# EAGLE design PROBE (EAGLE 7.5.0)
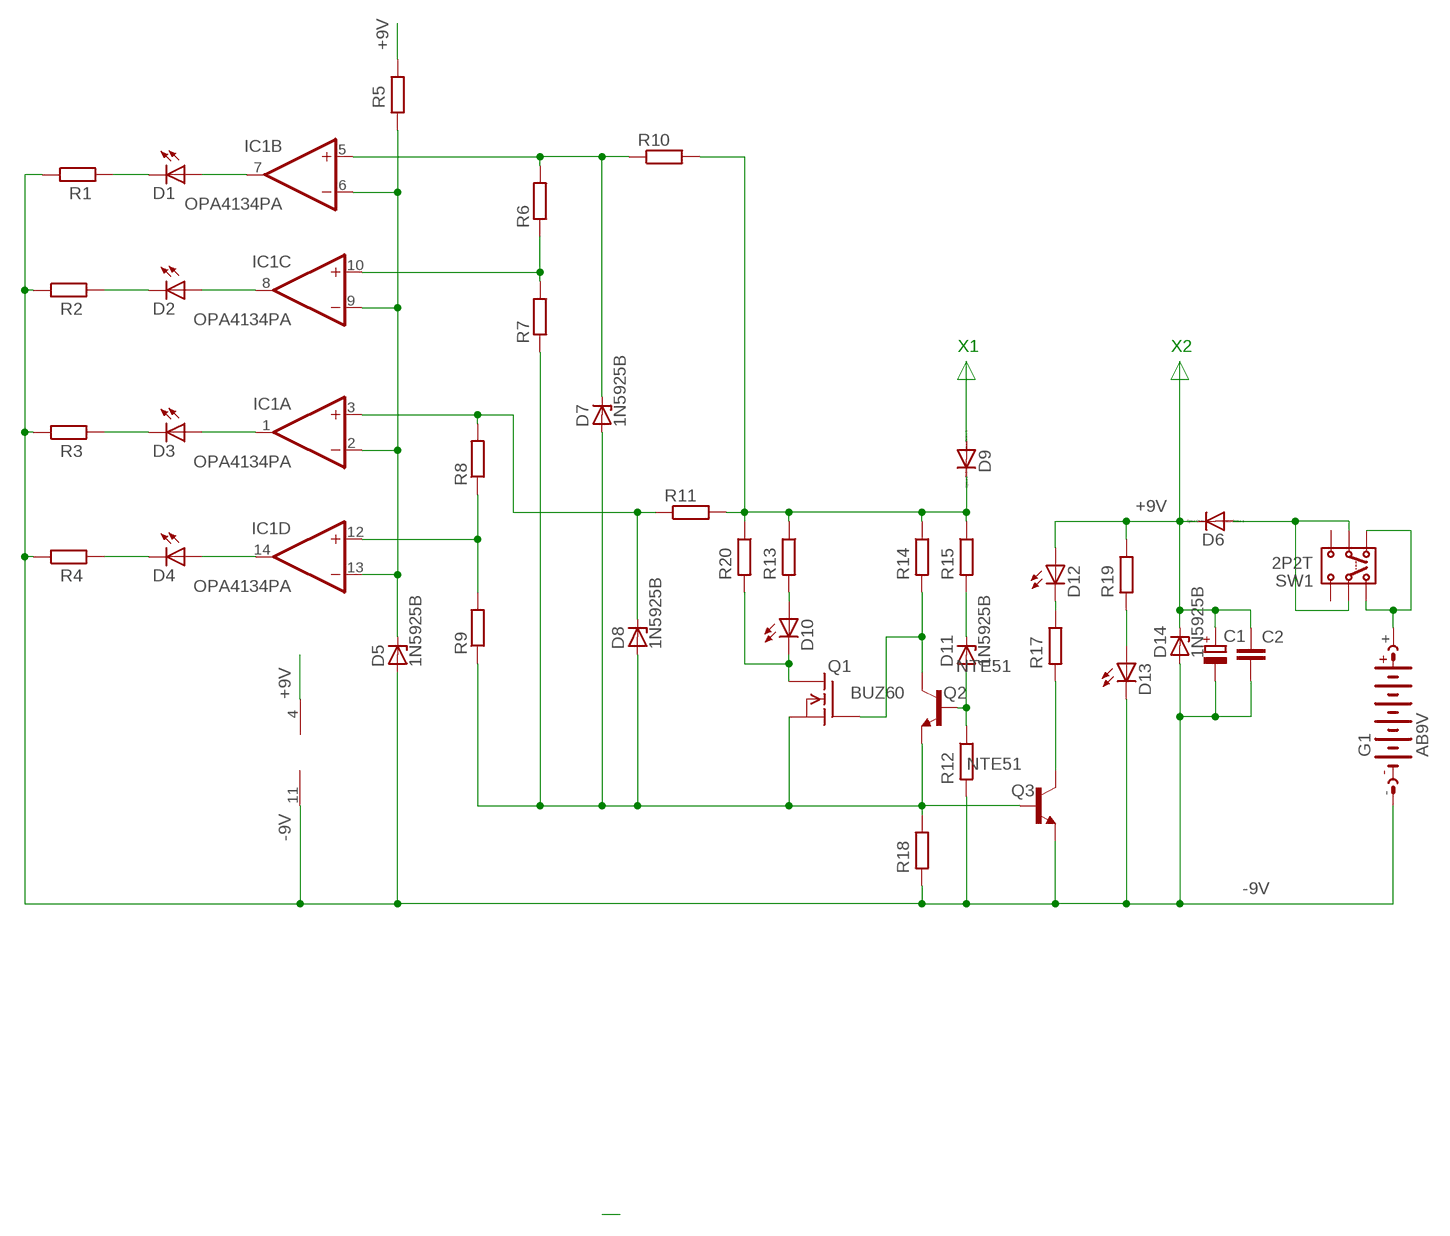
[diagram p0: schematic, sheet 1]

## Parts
C1  CPOL-EUE5-10.5  [E5-10,5]
C2  C-EUC1206  [C1206]
D1  LED5MM  [LED5MM]
D2  LED5MM  [LED5MM]
D3  LED5MM  [LED5MM]
D4  LED5MM  [LED5MM]
D5  1N5925B  BZX85  [DO41Z10]
D6  1N4004  [DO41-10]
D7  1N5925B  BZX85  [DO41Z10]
D8  1N5925B  BZX85  [DO41Z10]
D9  1N4004  [DO41-10]
D10  LED5MM  [LED5MM]
D11  1N5925B  BZX85  [DO41Z10]
D12  LED5MM  [LED5MM]
D13  LED5MM  [LED5MM]
D14  1N5925B  BZX85  [DO41Z10]
G1  AB9V  [AB9V]
IC1  OPA4134PA  [DIL14]
Q1  BUZ60  [TO220]
Q2  NTE51  2N5496  [TO220]
Q3  NTE51  2N5496  [TO220]
R1  R-EU_0204/7  [0204/7]
R2  R-EU_0204/7  [0204/7]
R3  R-EU_0204/7  [0204/7]
R4  R-EU_0204/7  [0204/7]
R5  R-EU_0204/7  [0204/7]
R6  R-EU_0204/7  [0204/7]
R7  R-EU_0204/7  [0204/7]
R8  R-EU_0204/7  [0204/7]
R9  R-EU_0204/7  [0204/7]
R10  R-EU_0617/22  [0617/22]
R11  R-EU_0617/22  [0617/22]
R12  R-EU_0204/7  [0204/7]
R13  R-EU_0204/7  [0204/7]
R14  R-EU_0204/7  [0204/7]
R15  R-EU_0204/7  [0204/7]
R17  R-EU_0204/7  [0204/7]
R18  R-EU_0204/7  [0204/7]
R19  R-EU_0204/7  [0204/7]
R20  R-EU_0204/7  [0204/7]
SW1  2P2T  [2P2T]

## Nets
+9V: C1.+ C2.1 D6.C D12.A D14.C IC1.4(P:V+) R5.1 R19.1
-9V: C1.- C2.2 D5.A D13.K(C) D14.A G1.- IC1.11(P:V-) Q3.3(E) R1.1 R2.1 R3.1 R4.1 R12.2 R18.2
N$1: D13.A R19.2
N$2: D11.A Q2.1(B) R12.1
N$3: D3.A IC1.1(A:OUT)
N$4: D12.K(C) R17.1
N$5: Q3.2(C) R17.2
N$6: D11.C R15.2
N$7: Q1.1(G) Q2.2(C) R14.2
N$9: D7.A D8.A Q1.3(S) Q2.3(E) Q3.1(B) R7.1 R9.1 R18.1
N$10: D10.K(C) Q1.2(D) R20.2
N$11: D10.A R13.2
N$12: D5.C IC1.2(A:-IN) IC1.6(B:-IN) IC1.9(C:-IN) IC1.13(D:-IN) R5.2
N$13: D9.C R10.2 R11.2 R13.1 R14.1 R15.1 R20.1
N$14: D8.C IC1.3(A:+IN) R8.2 R11.1
N$15: D7.C IC1.5(B:+IN) R6.2 R10.1
N$16: IC1.10(C:+IN) R6.1 R7.2
N$17: D1.A IC1.7(B:OUT)
N$18: IC1.12(D:+IN) R8.1 R9.2
N$19: D2.A IC1.8(C:OUT)
N$20: D4.A IC1.14(D:OUT)
N$21: D4.K(C) R4.2
N$22: D3.K(C) R3.2
N$23: G1.+ SW1.1.1 SW1.1.2
N$24: D2.K(C) R2.2
N$25: D6.A SW1.2.1 SW1.2.2
N$27: D1.K(C) R1.2
N$29: D9.A
Unconnected: SW1.3.1 SW1.3.2

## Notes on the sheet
- X1 | X2

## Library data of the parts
C1 = rcl:CPOL-EU: POLARIZED CAPACITOR, European symbol
C2 = rcl:C-EU: CAPACITOR, European symbol
D1-D4 D10 D12 D13 = led:LED: LED
D5 D7 D8 D11 D14 = diode:BZX85: Z DIODE
D6 D9 = diode:1N4004: DIODE
G1 = battery:AB9V: 9-V BATTERY CLIP
IC1 = linear:OPA4*: Quad Operational Amplifier compatible with: TLC27L4 Low Power, Single-Supply, Rail-To-Rail Operational Amplifier Source: http://focus.ti.com/lit/ds/symlink/opa2345.pdf http://focus.ti.com .. opa241.pdf http://focus.ti.com .. tlc27l4.pdf http://focus.ti.com/lit/ds/symlink/opa2134.pdf
Q1 = transistor-fet:BUZ60: N-Channel Enhancement MOSFET 400V; 5,5A; 1,0Ohm
Q2 Q3 = transistor-npn:2N5496: NPN Transistor
R1-R15 R17-R20 = rcl:R-EU_: RESISTOR, European symbol
SW1 = switch:2P2T: SLIDE SWITCH 2P2T Part No. SS-22F05-G(A)4 Source: CANAL ELECTRONIC CO., LTD .. switsch.pdf

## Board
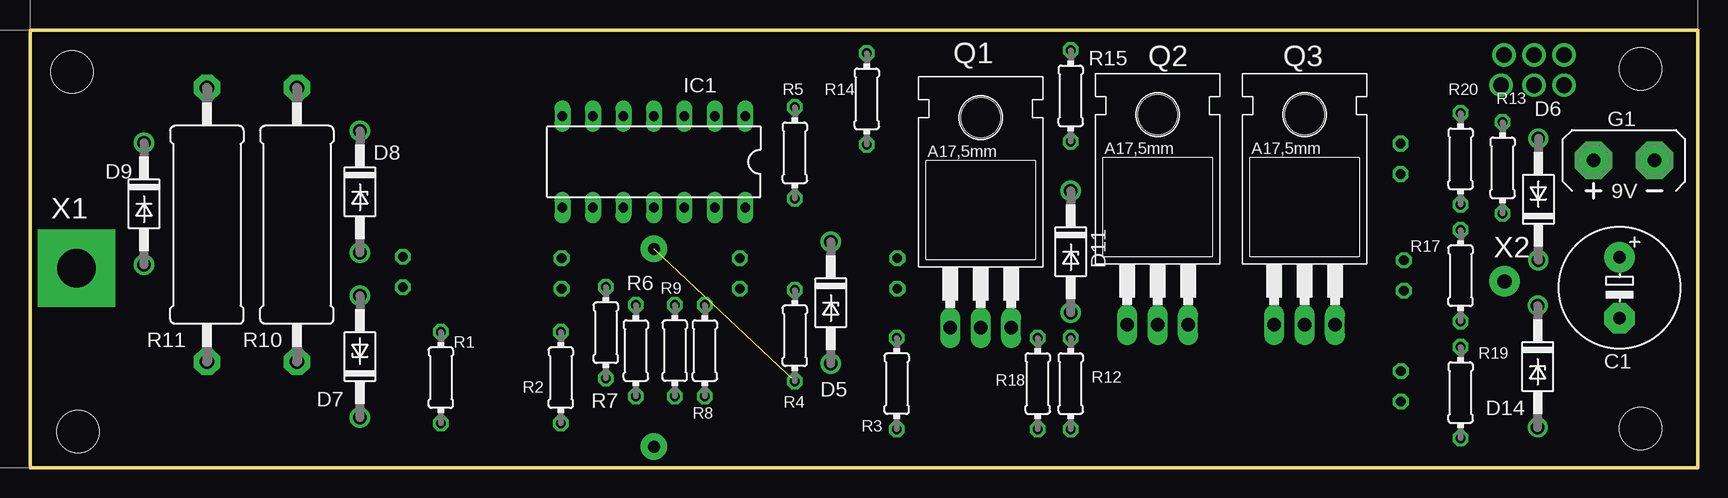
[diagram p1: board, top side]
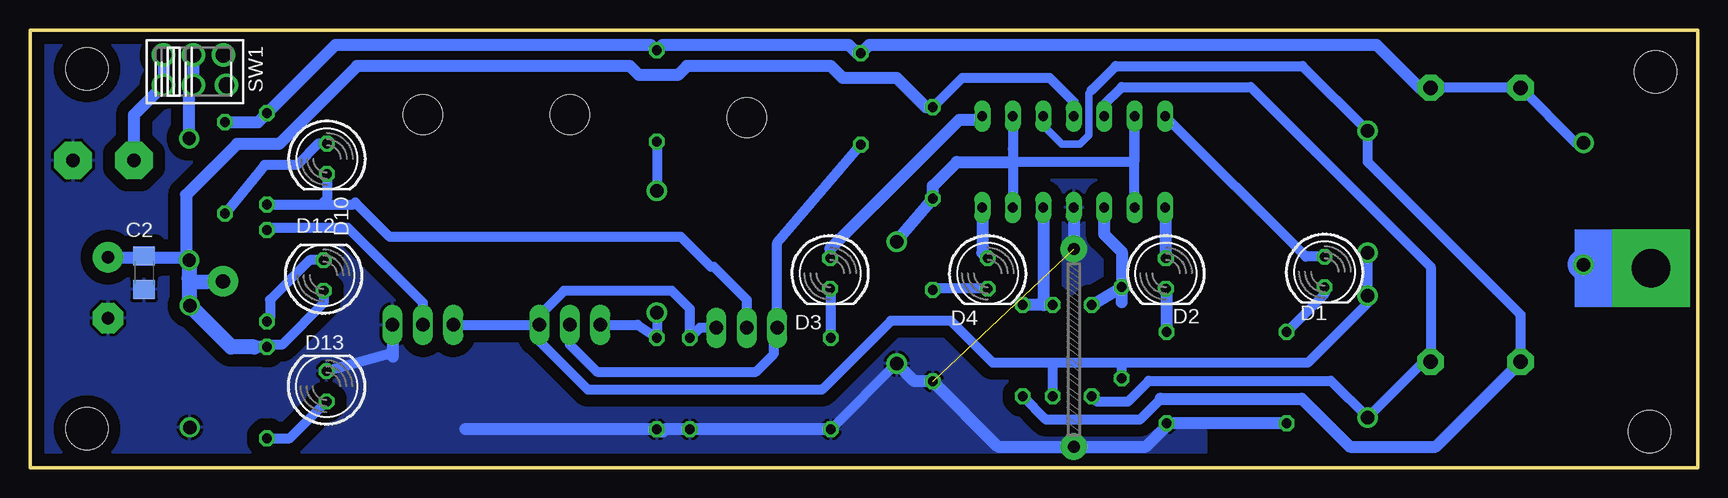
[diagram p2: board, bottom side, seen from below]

Size 139 x 36.5 mm. Coordinates in mm from the lower left corner, seen from the top.
Outline: 0,0 0,36.5 139,36.5 139,0 0,0
Copper layers (1*16): Top 0.035mm / dielectric 1.5mm / Bottom 0.035mm
Design rules "default": minimum track width 10mil, minimum drill 24mil, track to track 8mil, track to pad 8mil, pad to pad 8mil, via to via 8mil, smd to smd 8mil, copper to edge 40mil, drill to drill 8mil, minimum pad ring 10mil, minimum via ring 8mil, stop-mask expansion 4mil, vias tented up to drill 0mil, thermal gap 10mil
Holes 3.5 mm at 3.5,33 4,3 134.25,3.25 134.25,33.25

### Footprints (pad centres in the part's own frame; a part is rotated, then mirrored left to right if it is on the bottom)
E5-10,5 = drill 1.016 pad 2.54: + -2.54,0 | drill 1.016 pad 2.54 octagon: - 2.54,0
C1206 = smd 1.6 x 1.8: 1 -1.4,0; 2 1.4,0
LED5MM = drill 0.813 octagon: A -1.27,0; K 1.27,0
DO41Z10 = drill 1.118: A 5.08,0; C -5.08,0
DO41-10 = drill 1.118: A 5.08,0; C -5.08,0
AB9V = drill 1.118 pad 3.15 octagon: + 0,2.54; - 0,-2.54
DIL14 = drill 0.813 long: 1 -7.62,-3.81; 2 -5.08,-3.81; 3 -2.54,-3.81; 4 0,-3.81; 5 2.54,-3.81; 6 5.08,-3.81; 7 7.62,-3.81; 8 7.62,3.81; 9 5.08,3.81; 10 2.54,3.81; 11 0,3.81; 12 -2.54,3.81; 13 -5.08,3.81; 14 -7.62,3.81
TO220 = drill 1.118 long: 1 -2.54,-6.35; 2 0,-6.35; 3 2.54,-6.35 | hole 3.302: 0,11.176
0204/7 = drill 0.813 octagon: 1 -3.81,0; 2 3.81,0
0617/22 = drill 1.2 pad 2.184 octagon: 1 -11.43,0; 2 11.43,0
2P2T = drill 1.3 pad 1.93: 1.1 -2.492,1.38; 1.2 -2.492,-1.126; 2.1 0,1.38; 2.2 0,-1.126; 3.1 2.492,1.38; 3.2 2.746,-1.126

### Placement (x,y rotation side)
C1  132.5,15 270 top
C2  129.5,16.25 270 bottom
D1  31.08,16.32 270 bottom
D2  44.31,16.19 270 bottom
D3  72.3,16.19 270 bottom
D4  59.17,16.19 270 bottom
D5  66.75,13.75 270 top
D6  125.73,22.37 90 top
D7  27.5,9.25 90 top
D8  27.5,23 270 top
D9  9.5,22 270 top
D10  114.25,25.75 270 bottom
D11  86.75,18 270 top
D12  114.53,16.02 90 bottom
D13  114.28,6.78 90 bottom
D14  125.67,8.43 270 top
G1  132.87,25.62 90 top
IC1  52,25.5 180 top
Q1  79.25,18 0 top
Q2  94,18.25 0 top
Q3  106.25,18.25 0 top
R1  34.25,7.5 90 top
R2  44.25,7.5 90 top
R3  72.25,7 90 top
R4  63.75,11 90 top
R5  63.75,26.25 270 top
R6  50.5,9.75 270 top
R7  48,11.25 90 top
R8  56.25,9.75 270 top
R9  53.75,9.75 90 top
R10  22.25,20.25 90 top
R11  14.75,20.25 90 top
R12  86.75,7 270 top
R13  122.75,25 270 top
R14  69.75,30.75 270 top
R15  86.75,31 270 top
R17  119.25,16 90 top
R18  84,7 270 top
R19  119.25,6.25 270 top
R20  119.25,25.75 270 top
SW1  125.38,33.02 0 bottom

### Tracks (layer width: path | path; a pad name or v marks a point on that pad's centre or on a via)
+9V  (via drill 1.2 pad 2.54)
  Bottom 0.406: C2.1 132,17.65 132,17.54
  Bottom 0.813: IC1.4 52,30.5 54,32.5 61.31,32.5 R5.1 | D12.A 114.53,13.73 118,10.25 119.06,10.25 R19.1
  Bottom 1.016: R5.1 64.31,30.06 66.75,32.5 71.25,32.5 72.25,33.5 84.25,33.5 85,32.75 88.25,32.75 89,33.5 111.75,33.5 118.25,27 121.75,27 126,22.75 126,17.75 | 126,17.75 126,17.56 D6.C | R19.1 120.31,10.06 | C1.+ 132,17.54 126.21,17.54 126,17.75
  Bottom 1.27: D6.C 125.73,15.77 | 125.73,15.77 125.73,13.56 D14.C 122.23,10.06 120.31,10.06 | v122.9,15.52 125.41,15.45 125.73,15.77
-9V  (via drill 1 pad 2.18)  (1 unrouted)
  Bottom 0.813: D13.K 109.02,9.52 108.75,9.25 | D5.A 66.77,8.67 R3.1 | 52,18.75 v52,18.25
  Bottom 1.016: R1.1 R2.1 44.25,3.5 46,1.75 v52,1.75 58.31,1.75 R4.1 65.27,7.19 D5.A | 108.75,9.25 108.75,10.36 Q3.3 | R3.1 R18.2 86.06,3.19 86.25,3 86.56,3 R12.2 102.69,3.19 | IC1.11 52,18.75
  pour Bottom (isolate 1.016): 41.17,35.65 138.3,35.65 138.3,0.92 41,0.92 41,35.65
N$1
  Bottom 0.813: R19.2 117.34,2.44 D13.A
N$2
  Bottom 0.813: D11.A R12.1 88.34,11.9 Q2.1
N$3
  Bottom 0.813: D3.A 72.3,18.25 | 59.93,29 IC1.1
  Bottom 1.016: 59.93,29 61.55,29 72.3,18.25
N$4
  Bottom 0.813: D12.K 115.7,17.3 119,14 119,12.44 R17.1
N$5
  Bottom 0.813: Q3.2 106.25,13.75 112.5,20 119.06,20 R17.2
N$6
  Bottom 0.813: R15.2 D11.C
N$7
  Bottom 0.813: Q2.2 94,10.25 91.75,8 78.5,8 77,9.5 77,11.36 Q1.1 76.71,18.73 R14.2
N$9
  Bottom 0.813: D8.A D7.A 27.5,13.75 32.5,8.75 47.75,8.75 | Q3.1 Q2.3 | Q1.3 83.16,11.65 R18.1 84,13.25 85.5,14.75 94.5,14.75 96.75,12.5 96.75,12.11 Q2.3 | Q2.3 96.75,11.69 96.75,10.75 92.5,6.5 73,6.5 67.25,12.25 62.25,12.25 58.75,8.75 53.5,8.75 | 47.75,8.75 53.5,8.75 | R7.1 48,8.5 47.75,8.75 | R9.1 53.75,8.5 53.5,8.75
N$10
  Bottom 0.813: Q1.2 79.25,14 82,16.75 82.25,16.75 84.75,19.25 109.02,19.25 111.89,22.11 112.06,21.94 114.75,21.94 | R20.2 114.75,21.94 | D10.K 114.25,22.44 114.75,21.94
N$11
  Bottom 0.813: D10.A 114.98,27.02 116.75,25.25 119.44,25.25 R13.2
N$12
  Bottom 0.813: IC1.9 IC1.6 46.92,25.58 47,25.5 57.08,25.5 | 57.08,25.5 IC1.2 57.08,26.58 | 57.08,25.5 IC1.13
  Bottom 1.016: D5.C 66.75,18.94 R5.2 63.75,23.5 61.75,25.5 57.08,25.5
N$13
  Bottom 0.813: D9.C 10.15,27.08 R11.2 R10.2
  Bottom 1.016: R10.2 23.18,31.68 26.75,35.25 69.06,35.25 R14.1 70.06,34.56 70.75,35.25 86.31,35.25 R15.1 86.81,34.81 87.25,35.25 113.56,35.25 R20.1 120,28.81 R13.1
N$14
  Bottom 0.61: IC1.3 54.54,28.54 53,27 51.5,27 50.75,27.75 50.75,31.25 50.5,31.5
  Bottom 0.813: R11.1 14.75,12.75 27.5,25.5 D8.C 32.92,33.5 48.5,33.5 50.5,31.5 | 44.75,5.75 46.5,4 54.31,4 R8.2
  Bottom 1.016: 44.75,5.75 33,5.75 29,1.75 21.82,1.75 R11.1
N$15
  Bottom 0.813: IC1.5 49.46,30.29 48,31.75 37.25,31.75 22.25,16.75 R10.1 22.85,8.82 D7.C 30.58,7.25 45.75,7.25 47.5,5.5 50.06,5.5 R6.2
N$16
  Bottom 1.016: IC1.10 49.46,19.46 48,18 R7.2 | 48,13.81 R7.2 | R6.1 R7.2
N$17
  Bottom 0.813: D1.A 32.66,17.59 IC1.7
N$18
  Bottom 1.016: R9.2 54.5,13.56 | 54.5,13.56 R8.1 | IC1.12 54.54,13.6 54.5,13.56
N$19
  Bottom 1.016: D2.A 44.31,21.62 IC1.8
N$20
  Bottom 1.016: IC1.14 59.62,17.91 D4.A
N$21
  Bottom 0.813: D4.K 63.64,14.92 R4.2
N$22
  Bottom 0.813: R3.2 72.25,14.87 D3.K
N$23
  Bottom 1.016: SW1.1.1 SW1.1.2 130.33,29.44 G1.+
N$24
  Bottom 1.016: R2.2 44.25,14.86 D2.K
N$25
  Bottom 1.016: D6.A 125.73,31.54 SW1.2.2 SW1.2.1
N$27
  Bottom 0.813: D1.K 31.08,14.48 R1.2
N$28  (via drill 3.2 pad 6.45)
  other vias: 3.88,16.62
N$30
  Bottom 2.54: 9.57,16.93 4.07,16.93 4.07,16.32
(copper drawn outside any net)
  shapes: Bottom area x1

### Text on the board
tPlace: X1 | X2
